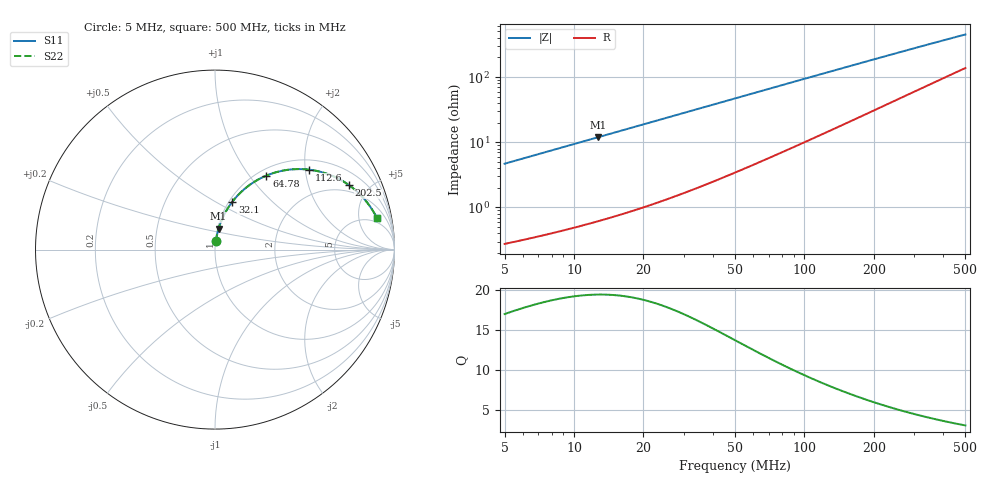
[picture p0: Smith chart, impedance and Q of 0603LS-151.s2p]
# MHz S MA R 50
!Freq  MagS11  AngS11  MagS21  AngS21  MagS12  AngS12  MagS22  AngS22
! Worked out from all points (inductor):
!   801 points, 5 MHz to 500 MHz, reference 50 ohm
!   read as one part in series: L = 149 nH near 5.116 MHz
!   highest Q = 19.4 at 12.7 MHz (marker M1), where L = 149 nH
!   S11 on the Smith chart (normalised r, x): 5 MHz: 1.01, +0.09; 32.1 MHz: 1.04, +0.60; 64.78 MHz: 1.10, +1.21; 112.6 MHz: 1.24, +2.10; 202.5 MHz: 1.63, +3.72; 500 MHz: 3.75, +8.57
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5  0.04665 84.0  0.9962 -2.7  0.9962 -2.7  0.04665 84.0
6.629336  0.06176 83.3  0.9947 -3.5  0.9947 -3.5  0.06176 83.3
8.345839  0.07762 82.5  0.9929 -4.4  0.9929 -4.4  0.07762 82.5
10.38652  0.09637 81.5  0.9904 -5.5  0.9904 -5.5  0.09637 81.5
12.70486  0.1175 80.3  0.987 -6.7  0.987 -6.7  0.1175 80.3
16.46152  0.1514 78.3  0.9806 -8.7  0.9806 -8.7  0.1514 78.3
20.9638  0.1911 75.9  0.9714 -11.0  0.9714 -11.0  0.1911 75.9
26.08976  0.2349 73.2  0.9588 -13.6  0.9588 -13.6  0.2349 73.2
32.09741  0.2841 70.1  0.9418 -16.5  0.9418 -16.5  0.2841 70.1
39.03642  0.3376 66.6  0.9196 -19.7  0.9196 -19.7  0.3376 66.6
46.66272  0.3919 63.0  0.8928 -23.0  0.8928 -23.0  0.3919 63.0
55.14041  0.4468 59.2  0.8612 -26.5  0.8612 -26.5  0.4468 59.2
64.78433  0.5022 55.2  0.8241 -30.0  0.8241 -30.0  0.5022 55.2
87.89618  0.6083 47.1  0.7361 -37.3  0.7361 -37.3  0.6083 47.1
112.5823  0.6883 40.3  0.6512 -43.1  0.6512 -43.1  0.6883 40.3
140.1103  0.7497 34.5  0.5711 -48.0  0.5711 -48.0  0.7497 34.5
170.4002  0.7956 29.6  0.4995 -51.9  0.4995 -51.9  0.7956 29.6
202.521  0.8288 25.7  0.439 -54.8  0.439 -54.8  0.8288 25.7
253.4954  0.8625 21.1  0.3667 -57.8  0.3667 -57.8  0.8625 21.1
336.1012  0.8925 16.3  0.2888 -60.2  0.2888 -60.2  0.8925 16.3
418.2828  0.9087 13.3  0.2387 -61.0  0.2387 -61.0  0.9087 13.3
500  0.9185 11.2  0.2041 -61.0  0.2041 -61.0  0.9185 11.2
